VAR_GLOBAL CONSTANT
	// Sampling
	cOversamples 		: UDINT 	:= 10;								// number of oversamples
	cSampleRate			: LREAL		:= 10000.0;							// Sample rate of input signal
	                                                                	
	// Resolution                                                   	
	cFFTLength			: UDINT		:= 512;								// length of FFT
	cFFTResult			: UDINT		:= cFFTLength / 2 + 1;
	cResolution			: LREAL		:= cSampleRate / cFFTLength;		// Reslution in frequency domain
	         
	// SDFT properties
	cBins				: UDINT		:= cFFTResult;						// Number of bins to be computed
	cDampingFactor		: LREAL		:= 0.999;							// Damping factor
END_VAR
